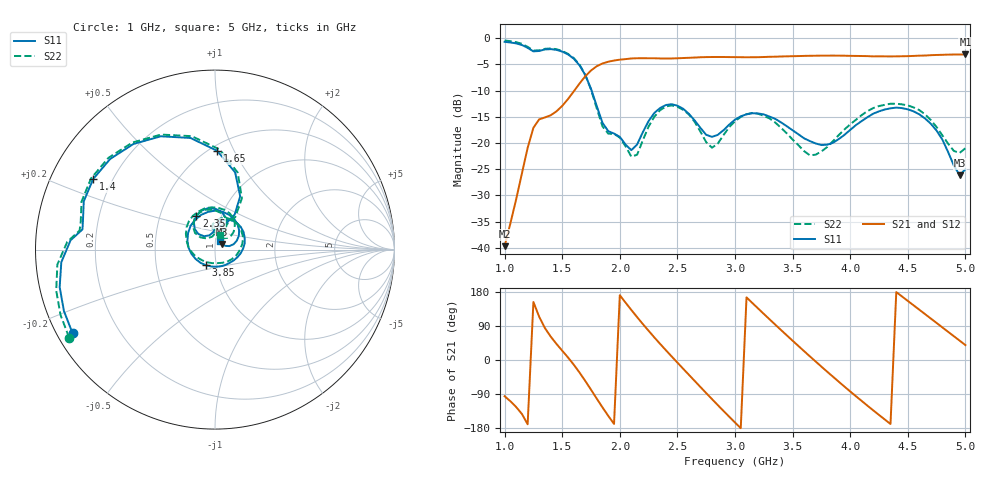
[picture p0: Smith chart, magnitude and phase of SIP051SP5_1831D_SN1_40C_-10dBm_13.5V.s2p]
# GHz  S  dB  R  50
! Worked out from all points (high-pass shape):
!   81 points, 1 GHz to 5 GHz, reference 50 ohm
!   highest |S21| = -3.12 dB at 5 GHz (marker M1); lowest = -39.7 dB at 1 GHz (marker M2)
!   |S21| within 3 dB of the highest: 1.754 GHz to end of sweep
!   lowest |S11| = -26.1 dB at 4.95 GHz (marker M3), VSWR 1.10, Z = 53.8 + j3.43 ohm
!   |S11| at or under -10 dB: 1.755 GHz to end of sweep
!   |S22| runs from -22.6 to -0.5 dB; largest |S21 - S12| = 0.0022
!   S11 on the Smith chart (normalised r, x): 1 GHz: 0.04, -0.27; 1.4 GHz: 0.13, +0.26; 1.65 GHz: 0.55, +0.86; 2.35 GHz: 0.76, +0.30; 3.85 GHz: 0.89, -0.16; 5 GHz: 1.05, +0.10
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1  -0.72 -149.6  -39.67 -95.6  -39.48 -95.6  -0.45 -148.9
1.25  -2.54 171.3  -17.10 153.1  -17.10 153.1  -2.36 172.0
1.4  -2.11 149.9  -14.72 61.8  -14.72 61.7  -1.98 150.1
1.65  -5.19 88.7  -8.67 -33.0  -8.67 -32.9  -5.05 87.4
1.7  -7.04 75.4  -7.29 -55.2  -7.30 -55.1  -6.98 73.6
1.85  -16.16 67.4  -4.83 -125.2  -4.83 -125.3  -16.85 67.1
2  -18.84 91.1  -4.12 171.0  -4.12 171.1  -18.98 89.1
2.2  -17.94 136.8  -3.84 94.9  -3.83 94.9  -19.48 140.0
2.35  -13.33 118.7  -3.88 42.5  -3.88 42.5  -13.75 124.0
2.5  -12.89 88.8  -3.85 -6.8  -3.85 -6.8  -13.10 91.6
2.7  -17.13 65.4  -3.65 -71.3  -3.67 -71.2  -17.84 63.0
2.8  -18.84 75.4  -3.61 -103.1  -3.62 -103.1  -20.91 80.0
3  -15.54 75.8  -3.63 -165.0  -3.63 -164.9  -15.85 88.3
3.15  -14.33 51.2  -3.65 150.6  -3.65 150.6  -14.28 58.9
3.35  -15.41 12.3  -3.55 93.1  -3.56 93.1  -16.12 12.3
3.7  -20.09 -68.3  -3.37 -3.9  -3.35 -4.0  -22.23 -103.3
3.85  -19.97 -119.6  -3.34 -44.0  -3.34 -44.1  -19.66 -152.5
4.1  -15.82 161.7  -3.42 -108.1  -3.41 -108.3  -14.67 151.5
4.35  -13.40 100.2  -3.50 -168.9  -3.50 -168.9  -12.52 104.0
4.7  -16.34 29.7  -3.26 109.3  -3.26 109.5  -15.64 48.3
4.95  -26.15 40.2  -3.13 51.1  -3.13 51.0  -21.90 61.2
5  -25.01 62.6  -3.12 39.4  -3.13 39.5  -21.02 70.8
